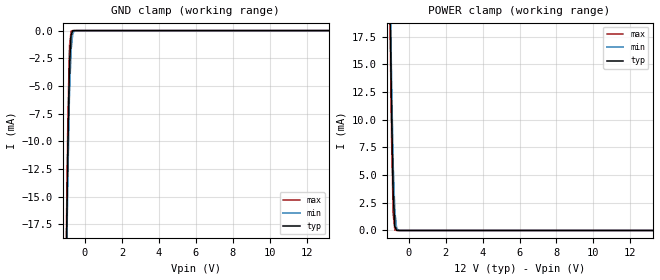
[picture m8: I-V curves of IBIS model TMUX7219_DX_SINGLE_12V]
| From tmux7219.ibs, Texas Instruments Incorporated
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[Model]   TMUX7219_DX_SINGLE_12V
Model_type   Terminator
|   typ   min   max
C_comp   62pF   62pF   62pF
[Voltage Range]   12   10.8   13.2
[Temperature Range]   27   125   -40
[Power Clamp Reference]   12   10.8   13.2
[GND Clamp Reference]   0   0   0
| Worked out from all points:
|   GND clamp passes 1 mA (typ) near -0.77 V on its own axis
|   POWER clamp passes 1 mA (typ) near -0.77 V on its own axis
[GND Clamp]
|   Voltage   I(typ)   I(min)   I(max)
-30V      -4.646A    -4.64A     -4.649A
-1.02V    -22.01mA   -24.41mA   -19.81mA
-930mV    -11.04mA   -13.89mA   -8.565mA
-840mV    -3.269mA   -5.934mA   -1.414mA
-750mV    -384.6uA   -1.761mA   -36.1uA
-660mV    -13.98uA   -270.8uA   -466.8nA
-570mV    -397.4nA   -19.97uA   -233.4nA
-210mV    0A         0A         0A
60V       0A         0A         0A
[POWER Clamp]
|   Voltage   I(typ)   I(min)   I(max)
-30V      4.646A     4.64A      4.649A
-1.02V    22.01mA    24.41mA    19.81mA
-930mV    11.04mA    13.89mA    8.565mA
-840mV    3.269mA    5.934mA    1.414mA
-750mV    384.6uA    1.761mA    36.1uA
-660mV    13.98uA    270.8uA    466.8nA
-570mV    397.4nA    19.97uA    233.4nA
-210mV    0A         0A         0A
60V       0A         0A         0A
